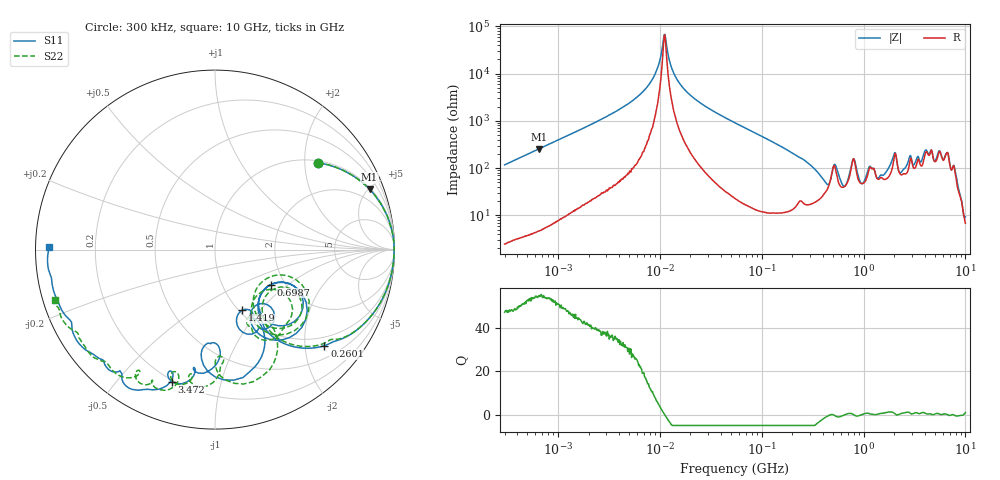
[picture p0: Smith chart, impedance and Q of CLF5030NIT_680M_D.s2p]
! S-Parameter Data Generated by TDK Corporation
! Copyright(C) 2019 TDK Corporation.
! All Rights Reserved.
! TDK P/N: CLF5030NIT-680M-D (Inductor)
! Property: L=68uH at 100kHz
! Size(LxWxT): 5.3x5x2.7mm
! Model Type: s2p (Touchstone File Format Version 1.0)
! Frequency: DC=Yes Start=0.3MHz Stop=10000MHz 802points Log-sweep
! Model Generated on May 10, 2019
! Port Assignments:
!  1 ---@@@--- 2
! Applicable Conditions:
!  Temperature = 25 degC
!  DC Bias Current = 0 A
!  Small Signal Operation
! Terms and conditions regarding TDK Simulation Models
! (1)This simulation model is being provided solely for informational purposes. Please refer to the specifications of the products in terms of detailed characteristics of such products.
! (2)In no event shall TDK Corporation of any of its subsidiaries be liable for any loss or damage arising, directly or indirectly,
!  From any information contained in this simulation model, including, but not limited to loss or damages arising from any inaccuracies, omissions or errors in connection with such information.
! (3)Any and all copyrights on this simulation model are owned by TDK Corporation.
!  Duplication or redistribution of this simulation model without prior written permission from TDK Corporation is prohibited.
! (4)This simulation model is subject to any modification or change without any prior notice.
! (5)Neither TDK Corporation nor any of its subsidiaries shall make any warranty, express or implied,
!  Including but not limited to the correctness, implied warranties of merchantability and fitness for a particular purpose with respect to this simulation models.
! (6)The use of this simulation model shall be deemed to have consented to the terms and conditions hereof.
# Hz S MA R 50
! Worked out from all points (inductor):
!   801 points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, 300 kHz to 10 GHz, reference 50 ohm
!   read as one part in series: L = 61.9 uH near 318.3 kHz
!   highest Q = 54.5 at 654.3 kHz (marker M1), where L = 61.8 uH
!   self-resonance near 11.09 MHz
!   S11 on the Smith chart (normalised r, x): 300 kHz: 1.05, +2.34; 260.1 MHz: 0.78, -2.44; 698.7 MHz: 1.69, -0.76; 1.419 GHz: 1.03, -0.81; 3.472 GHz: 0.19, -0.71; 10 GHz: 0.04, +0.01
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300000  0.7524 40.0  0.6432 -48.8  0.6432 -48.8  0.7521 40.0
654279  0.9245 21.3  0.3637 -67.7  0.3637 -67.7  0.9248 21.3
1713600  0.9857 8.4  0.1467 -80.3  0.1468 -80.3  0.9858 8.4
5955893  0.9982 1.6  0.0317 -86.2  0.03172 -86.2  0.9983 1.6
9671944  0.9986 -0.0  0.006883 -78.6  0.006899 -78.7  0.9986 -0.0
1.125452e7  0.9986 -0.5  0.001486 14.6  0.001494 14.5  0.9986 -0.5
1.35567e7  0.9984 -1.1  0.009263 79.2  0.009236 79.3  0.9984 -1.1
1.717743e7  0.9981 -1.9  0.02074 83.5  0.02075 83.5  0.9982 -1.9
5.477226e7  0.9912 -8.5  0.109 80.1  0.109 80.1  0.9913 -8.5
2.600778e8  0.811 -41.3  0.5053 42.8  0.5053 42.8  0.8037 -40.3
3.126428e8  0.7182 -49.5  0.5973 32.5  0.5973 32.5  0.7183 -48.5
4.20949e8  0.4445 -56.1  0.6985 6.2  0.6986 6.2  0.4542 -53.9
6.987102e8  0.3671 -32.0  0.6464 -26.7  0.6465 -26.7  0.3286 -29.6
8.528959e8  0.6067 -56.3  0.4741 -8.4  0.4743 -8.4  0.5987 -52.6
1.054047e9  0.4049 -48.0  0.6037 -41.7  0.6043 -41.7  0.3603 -39.0
1.418928e9  0.3701 -66.2  0.5559 -48.8  0.5567 -48.9  0.4788 -64.7
1.767019e9  0.5126 -59.0  0.4894 -80.6  0.4893 -80.7  0.5126 -53.2
2.08171e9  0.7277 -86.1  0.2317 -67.3  0.231 -67.6  0.7657 -78.0
2.416286e9  0.5241 -93.0  0.3934 -87.4  0.3922 -87.4  0.6027 -85.9
3.472057e9  0.7739 -108.2  0.1681 -110.7  0.1675 -110.6  0.7667 -108.3
6.495326e9  0.8933 -139.0  0.0542 -134.6  0.05419 -133.8  0.9072 -140.0
1e10  0.9263 179.2  0.06919 -92.7  0.06904 -92.8  0.9329 -162.6
